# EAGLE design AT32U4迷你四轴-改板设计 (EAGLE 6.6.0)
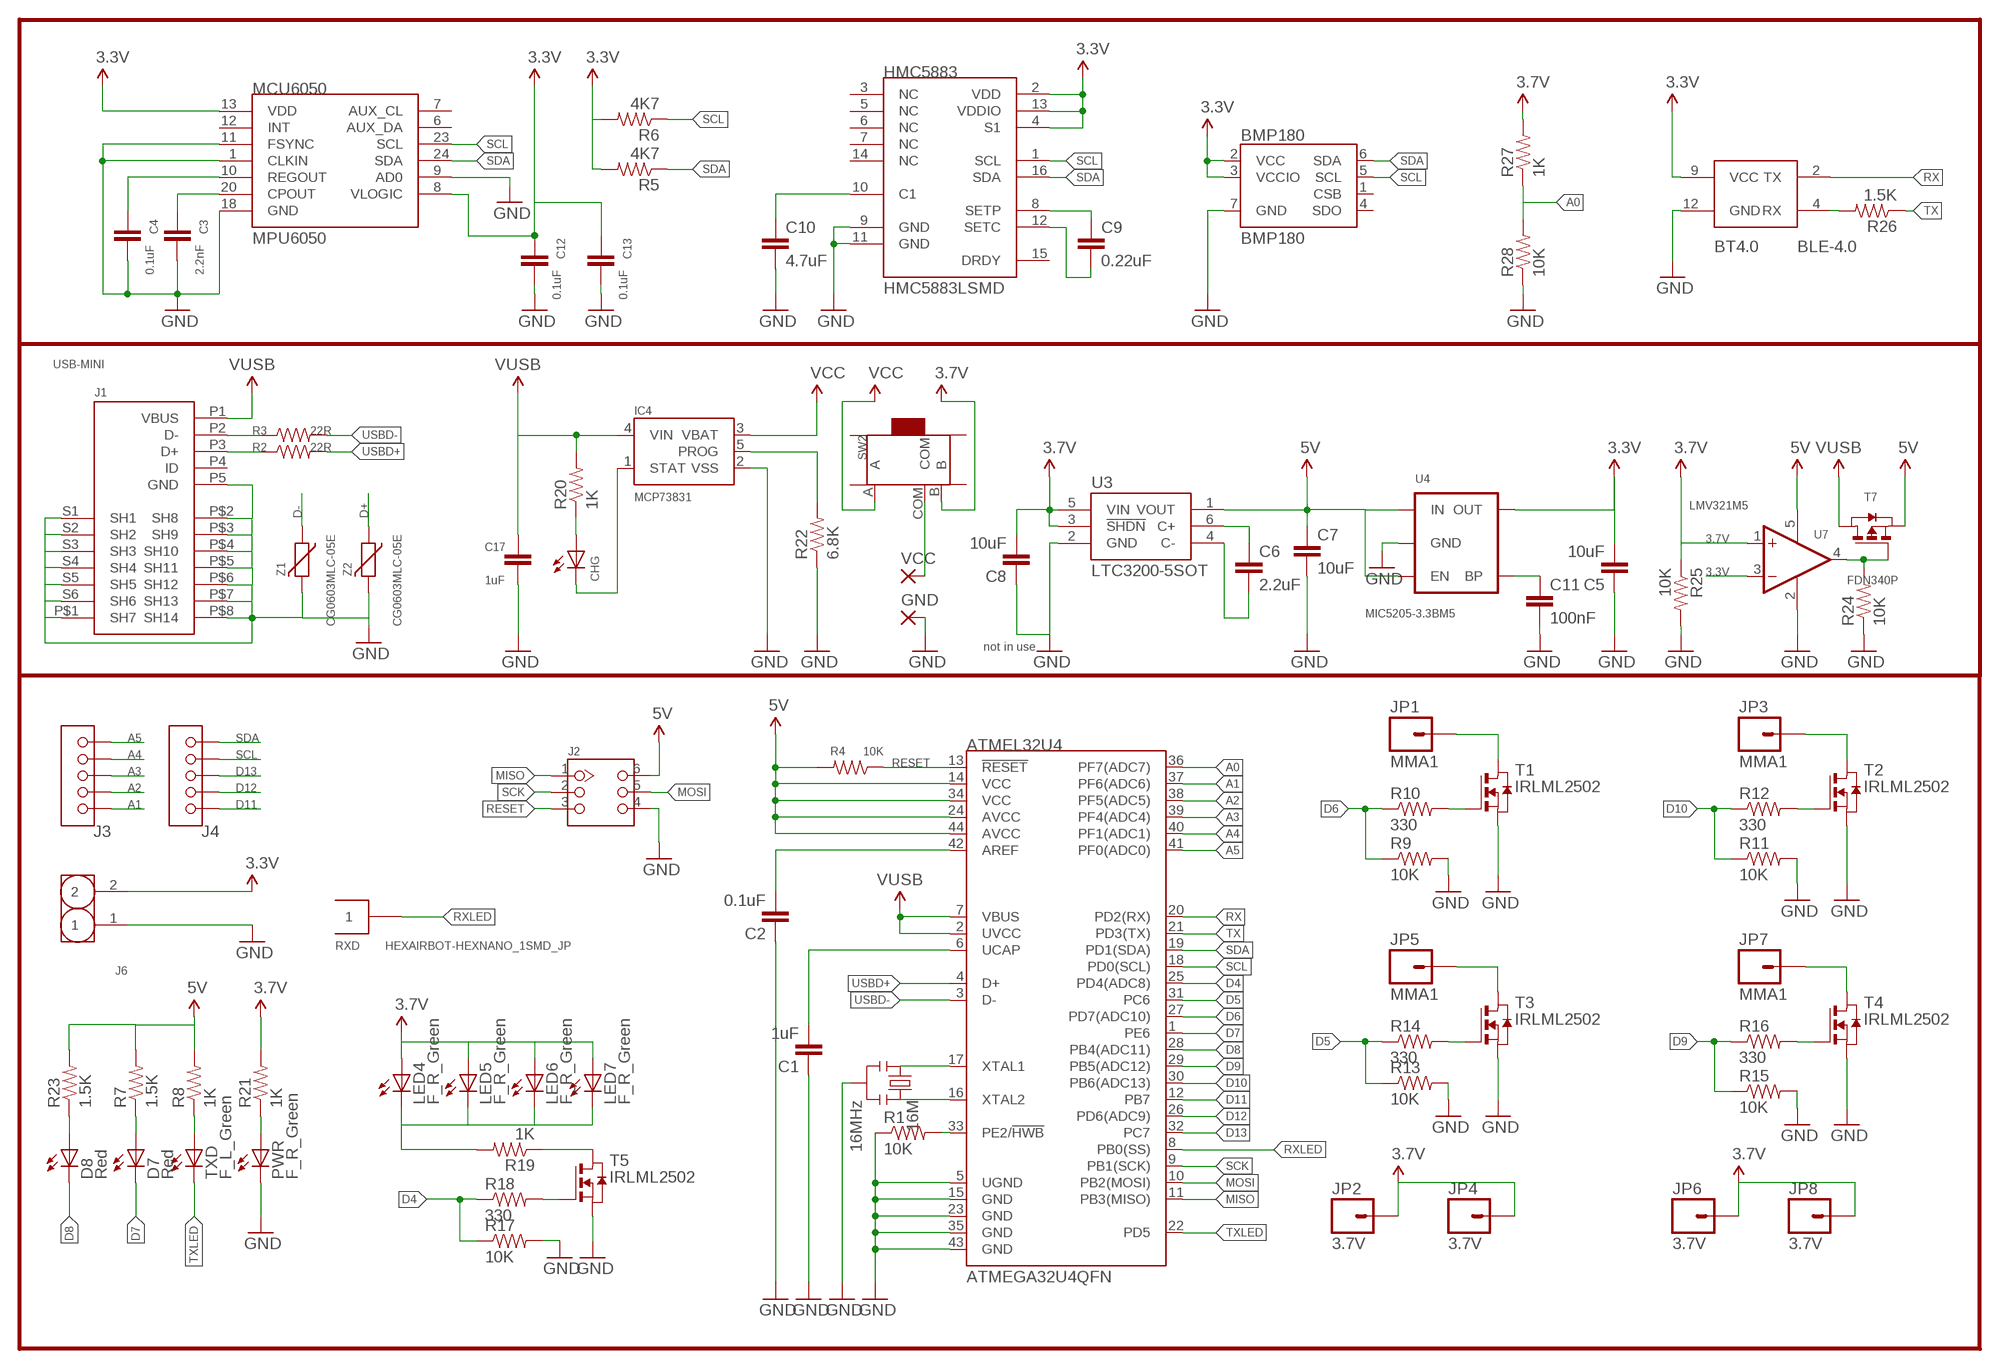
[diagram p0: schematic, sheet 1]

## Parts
16M  16MHz  RESONATOR16MHZ  [RESONATOR-SMD]
ATMEL32U4  ATMEGA32U4QFN  [SPARKFUN-DIGITALIC_QFN-44]
BMP180  BMP180  [BMP180]
BT4.0  BLE-4.0  HEXAIRBOT-HEXNANO_BLUETOOTH_HM11  [HEXAIRBOT-HEXNANO_BLUETOOTH_HM11]
C1  1uF  CAP0402-CAP  [0402-CAP]
C2  0.1uF  CAP0402-CAP  [0402-CAP]
C3  2.2nF  CAP0402-CAP  [0402-CAP]
C4  0.1uF  CAP0402-CAP  [0402-CAP]
C5  10uF  CAP0402-CAP  [0402-CAP]
C6  2.2uF  CAP0603-CAP  [0603-CAP]
C7  10uF  CAP0603-CAP  [0603-CAP]
C8  10uF  CAP0805  [0805]
C9  0.22uF  CAP0402-CAP  [0402-CAP]
C10  4.7uF  CAP0402-CAP  [0402-CAP]
C11  100nF  CAP0603-CAP  [0603-CAP]
C12  0.1uF  CAP0402-CAP  [0402-CAP]
C13  0.1uF  CAP0402-CAP  [0402-CAP]
C17  1uF  CAP0805  [0805]
CHG  Yellow  LEDCHIPLED_0603  [CHIPLED_0603]
D7  Red  LEDCHIPLED_0603  [CHIPLED_0603]
D8  Red  LEDCHIPLED_0603  [CHIPLED_0603]
GND  2,15/1,0  [2,15/1,0]
HMC5883  HMC5883LSMD  [16LPCC]
IC4  MCP73831  [SOT23-5]
J1  USB-MINI  [USB_MICRO]
J2  HEADER-2X3P-2.0  [2X3P-2.0]
J3  HEADER-5P-2.0  [5P-2.0]
J4  HEADER-5P-2.0  [5P-2.0]
J6  HEADER-2P-2.0  [2P-2.0]
JP1  MMA1  M01SMD-4.5X1.5  [PAD-1.5X4.5]
JP2  3.7V  M01SMD-4.5X1.5  [PAD-1.5X4.5]
JP3  MMA1  M01SMD-4.5X1.5  [PAD-1.5X4.5]
JP4  3.7V  M01SMD-4.5X1.5  [PAD-1.5X4.5]
JP5  MMA1  M01SMD-4.5X1.5  [PAD-1.5X4.5]
JP6  3.7V  M01SMD-4.5X1.5  [PAD-1.5X4.5]
JP7  MMA1  M01SMD-4.5X1.5  [PAD-1.5X4.5]
JP8  3.7V  M01SMD-4.5X1.5  [PAD-1.5X4.5]
LED4  F_R_Green  LEDCHIPLED_0603  [CHIPLED_0603]
LED5  F_R_Green  LEDCHIPLED_0603  [CHIPLED_0603]
LED6  F_R_Green  LEDCHIPLED_0603  [CHIPLED_0603]
LED7  F_R_Green  LEDCHIPLED_0603  [CHIPLED_0603]
MCU6050  MPU6050  TESTING_MPU-6050-1  [TESTING_QFN-24-4MM2]
PWR  F_R_Green  LEDCHIPLED_0603  [CHIPLED_0603]
R1  10K  RESISTOR0402-RES  [0402-RES]
R2  22R  RESISTOR0402-RES  [0402-RES]
R3  22R  RESISTOR0402-RES  [0402-RES]
R4  10K  RESISTOR0402-RES  [0402-RES]
R5  4K7  RESISTOR0402-RES  [0402-RES]
R6  4K7  RESISTOR0402-RES  [0402-RES]
R7  1.5K  RESISTOR0402-RES  [0402-RES]
R8  1K  RESISTOR0402-RES  [0402-RES]
R9  10K  RESISTOR0402-RES  [0402-RES]
R10  330  RESISTOR0402-RES  [0402-RES]
R11  10K  RESISTOR0402-RES  [0402-RES]
R12  330  RESISTOR0402-RES  [0402-RES]
R13  10K  RESISTOR0402-RES  [0402-RES]
R14  330  RESISTOR0402-RES  [0402-RES]
R15  10K  RESISTOR0402-RES  [0402-RES]
R16  330  RESISTOR0402-RES  [0402-RES]
R17  10K  RESISTOR0402-RES  [0402-RES]
R18  330  RESISTOR0402-RES  [0402-RES]
R19  1K  RESISTOR0402-RES  [0402-RES]
R20  1K  RESISTOR0402-RES  [0402-RES]
R21  1K  RESISTOR0402-RES  [0402-RES]
R22  6.8K  RESISTOR0402-RES  [0402-RES]
R23  1.5K  RESISTOR0402-RES  [0402-RES]
R24  10K  RESISTOR0402-RES  [0402-RES]
R25  10K  RESISTOR0402-RES  [0402-RES]
R26  1.5K  RESISTOR0402-RES  [0402-RES]
R27  1K  RESISTOR0402-RES  [0402-RES]
R28  10K  RESISTOR0402-RES  [0402-RES]
RXD  HEXAIRBOT-HEXNANO_1SMD_JP  [HEXAIRBOT-HEXNANO_1SMD]
SW2  SWITCH-3P-SMD-6.6X2.8  [3P-SMD-2CH-6.6X2.8-REINFORCE]
T1  IRLML2502  NMOSSOT23  [SOT-23]
T2  IRLML2502  NMOSSOT23  [SOT-23]
T3  IRLML2502  NMOSSOT23  [SOT-23]
T4  IRLML2502  NMOSSOT23  [SOT-23]
T5  IRLML2502  NMOSSOT23  [SOT-23]
T7  FDN340P  [SOT23]
TXD  F_L_Green  LEDCHIPLED_0603  [CHIPLED_0603]
U3  LTC3200-5SOT  [SOT23-6]
U4  MIC5205-3.3BM5  MIC52053.3V  [SOT23-5]
U7  LMV321M5  [SOT23-5]
VCC  2,15/1,0  [2,15/1,0]
Z1  CG0603MLC-05E  VARISTORCN0603  [CT/CN0603]
Z2  CG0603MLC-05E  VARISTORCN0603  [CT/CN0603]

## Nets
3.3V: BMP180.2(VCC) BMP180.3(VCCIO) BT4.0.9(VCC) C5.2 C12.1 C13.1 HMC5883.2(VDD) HMC5883.4(S1) HMC5883.13(VDDIO) J6.2 MCU6050.8(VLOGIC) MCU6050.13(VDD) R5.2 R6.2 U4.5(OUT) U7.3(-IN)
3.7V: C8.2 JP2.P$1 JP4.P$1 JP6.P$1 JP8.P$1 LED4.A LED5.A LED6.A LED7.A R21.2 R25.1 R27.2 SW2.B U3.3(!SHDN) U3.5(VIN) U7.1(+IN)
5V: ATMEL32U4.14(VCC) ATMEL32U4.24(AVCC) ATMEL32U4.34(VCC) ATMEL32U4.44(AVCC) C7.1 J2.6 R4.2 R7.2 R8.2 R23.2 T7.2(S) U3.1(VOUT) U4.1(IN) U4.3(EN) U7.5(V+)
A0: ATMEL32U4.36(PF7(ADC7)) R27.1 R28.2
A1: ATMEL32U4.37(PF6(ADC6)) J3.1
A2: ATMEL32U4.38(PF5(ADC5)) J3.2
A3: ATMEL32U4.39(PF4(ADC4)) J3.3
A4: ATMEL32U4.40(PF1(ADC1)) J3.4
A5: ATMEL32U4.41(PF0(ADC0)) J3.5
D4: ATMEL32U4.25(PD4(ADC8)) R17.1 R18.1
D5: ATMEL32U4.31(PC6) R13.1 R14.1
D6: ATMEL32U4.27(PD7(ADC10)) R9.1 R10.1
D7: ATMEL32U4.1(PE6) D7.C
D8: ATMEL32U4.28(PB4(ADC11)) D8.C
D9: ATMEL32U4.29(PB5(ADC12)) R15.1 R16.1
D10: ATMEL32U4.30(PB6(ADC13)) R11.1 R12.1
D11: ATMEL32U4.12(PB7) J4.1
D12: ATMEL32U4.26(PD6(ADC9)) J4.2
D13: ATMEL32U4.32(PC7) J4.3
D+: J1.P3(D+) R2.1 Z2.1
D-: J1.P2(D-) R3.1 Z1.1
GND: 16M.2 ATMEL32U4.5(UGND) ATMEL32U4.15(GND) ATMEL32U4.23(GND) ATMEL32U4.35(GND) ATMEL32U4.43(GND) BMP180.7(GND) BT4.0.12(GND) C1.1 C2.1 C3.2 C4.2 C5.1 C7.2 C8.1 C10.2 C11.2 C12.2 C13.2 C17.1 GND.1(P) HMC5883.9(GND) HMC5883.11(GND) IC4.2(VSS) J1.P5(GND) J1.P$1(SH7) J1.P$2(SH8) J1.P$3(SH9) J1.P$4(SH10) J1.P$5(SH11) J1.P$6(SH12) J1.P$7(SH13) J1.P$8(SH14) J1.S1(SH1) J1.S2(SH2) J1.S3(SH3) J1.S4(SH4) J1.S5(SH5) J1.S6(SH6) J2.4 J6.1 MCU6050.1(CLKIN) MCU6050.9(AD0) MCU6050.11(FSYNC) MCU6050.18(GND) PWR.C R1.1 R9.2 R11.2 R13.2 R15.2 R17.2 R22.1 R24.1 R25.2 R28.1 T1.2(S) T2.2(S) T3.2(S) T4.2(S) T5.2(S) U3.2(GND) U4.2(GND) U7.2(V-) Z1.2 Z2.2
MISO: ATMEL32U4.11(PB3(MISO)) J2.1
MOSI: ATMEL32U4.10(PB2(MOSI)) J2.5
N$1: 16M.1 ATMEL32U4.17(XTAL1)
N$2: 16M.3 ATMEL32U4.16(XTAL2)
N$3: CHG.C IC4.1(STAT)
N$4: CHG.A R20.1
N$5: ATMEL32U4.6(UCAP) C1.2
N$6: ATMEL32U4.42(AREF) C2.2
N$7: R8.1 TXD.A
N$8: C4.1 MCU6050.10(REGOUT)
N$9: C3.1 MCU6050.20(CPOUT)
N$10: D7.A R7.1
N$11: ATMEL32U4.33(PE2/!HWB) R1.2
N$12: R18.2 T5.3(G)
N$13: PWR.A R21.1
N$14: R12.2 T2.3(G)
N$15: R10.2 T1.3(G)
N$16: JP1.P$1 T1.1(D)
N$17: JP3.P$1 T2.1(D)
N$18: R14.2 T3.3(G)
N$19: JP5.P$1 T3.1(D)
N$20: R16.2 T4.3(G)
N$21: JP7.P$1 T4.1(D)
N$22: R19.1 T5.1(D)
N$23: C9.1 HMC5883.8(SETP)
N$24: LED4.C LED5.C LED6.C LED7.C R19.2
N$25: C6.1 U3.6(C+)
N$26: IC4.5(PROG) R22.2
N$27: C6.2 U3.4(C-)
N$28: C9.2 HMC5883.12(SETC)
N$29: C10.1 HMC5883.10(C1)
N$30: SW2.COM VCC.1(P)
N$31: C11.1 U4.4(BP)
N$32: D8.A R23.1
N$34: R24.2 T7.3(G) U7.4(OUT)
N$35: BT4.0.4(RX) R26.2
RESET: ATMEL32U4.13(!RESET) J2.3 R4.1
RX: ATMEL32U4.20(PD2(RX)) BT4.0.2(TX)
RXLED: ATMEL32U4.8(PB0(SS)) RXD.1
SCK: ATMEL32U4.9(PB1(SCK)) J2.2
SCL: ATMEL32U4.18(PD0(SCL)) BMP180.5(SCL) HMC5883.1(SCL) J4.4 MCU6050.23(SCL) R6.1
SDA: ATMEL32U4.19(PD1(SDA)) BMP180.6(SDA) HMC5883.16(SDA) J4.5 MCU6050.24(SDA) R5.1
TX: ATMEL32U4.21(PD3(TX)) R26.1
TXLED: ATMEL32U4.22(PD5) TXD.C
USBD+: ATMEL32U4.4(D+) R2.2
USBD-: ATMEL32U4.3(D-) R3.2
VCC: IC4.3(VBAT) SW2.A
VUSB: ATMEL32U4.2(UVCC) ATMEL32U4.7(VBUS) C17.2 IC4.4(VIN) J1.P1(VBUS) R20.2 T7.1(D)
Unconnected: BMP180.1(CSB) BMP180.4(SDO) HMC5883.3(NC) HMC5883.5(NC) HMC5883.6(NC) HMC5883.7(NC) HMC5883.14(NC) HMC5883.15(DRDY) J1.P4(ID) MCU6050.6(AUX_DA) MCU6050.7(AUX_CL) MCU6050.12(INT) SW2.SS1 SW2.SS2 SW2.SS3 SW2.SS4

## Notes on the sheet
- not in use

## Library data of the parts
16M = SparkFun-FreqCtrl:RESONATOR: Resonator Small SMD resonator. Used, eg, on the Arduino Pro/ Pro Mini boards. 8MHz- XTAL-08895 16MHz- XTAL-08900; PROD_ID: XTAL-08900
ATMEL32U4 = SparkFun-DigitalIC:ATMEGA32U4: Atmel 44-pin 8-bit Microcontroller with 32KBytes of ISP Flash and USB Controller ----- Please use the QFN-44-NOPAD_1:1 package for the footprint of all boards using a 32U4. Route traces directly away from the pads as much as possible.
BMP180 = duinofun-ic:BMP180: BMP085 Pressure Sensor Great little MEMS pressure sensor. SKU: COM-09603
BT4.0 = MainBoard:HEXAIRBOT-HEXNANO_BLUETOOTH_HM11: BLE 4.0 Module
C1-C13 = SparkFun-Passives:CAP: Capacitor
C17 = SparkFun:CAP: Capacitor
CHG D7 D8 LED4-LED7 PWR TXD = led:LED: LED
GND VCC = wirepad:2,15/1,0: THROUGH-HOLE PAD
HMC5883 = HexAirbot-HexNano:HMC5883L: 3 Axis Digital Compass IC
IC4 = SparkFun:MCP73831: Microchip's MCP73831 Miniature single cell, fully integrated Li-Ion, Li-polymer charge management controller http://ww1.microchip.com/downloads/en/DeviceDoc/21984a.pdf
J1 = QXZ:USB-MINI
J2 = SeeedStudio-Connector:HEADER-2X3P
J3 J4 = SeeedStudio-Connector:HEADER-5P
J6 = SeeedStudio-Connector:HEADER-2P
JP1-JP8 = SparkFun-Connectors:M01: Header 1
MCU6050 = MPU6050:TESTING_MPU-6050
R1-R28 = SparkFun-Passives:RESISTOR: Resistor
RXD = MainBoard:HEXAIRBOT-HEXNANO_1SMD_JP
SW2 = duinofun-ic:SWITCH-3P-SMD
T1-T5 = zetex:NMOSSOT23: MOS FET; OC_FARNELL: unknown; OC_NEWARK: unknown
T7 = HexAirbot-HexNano:FDN340P: MOS FET
U3 = HexAirbot-HexNano:LTC3200-5: Linear Technology. Low Noise, Regulated Charge Pump DC/DC Converters, SOT23-6. Fixed 5V ± 4% Output or ADJ VIN Range: 2.7V to 4.5V
U4 = SparkFun-PowerIC:MIC5205: MIC5205 150mA vreg 3.3V - VREG-00822 5V - VREG-00823; PROD_ID: VREG-00822
U7 = linear:LMV321?*: General Purpose, Low Voltage, Rail-to-Rail Output Operational Amplifiers Source: http://www.national.com/mpf/LM/LMV321.html http://www.national.com/dt/lmv_qual.pdf
Z1 Z2 = varistor:VARISTOR: VARISTOR

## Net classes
0 default: width 0.254 mm, drill 0.61 mm, clearance 0.254 mm
2 gnd: width 0.254 mm, drill 0.61 mm, clearance 0.254 mm

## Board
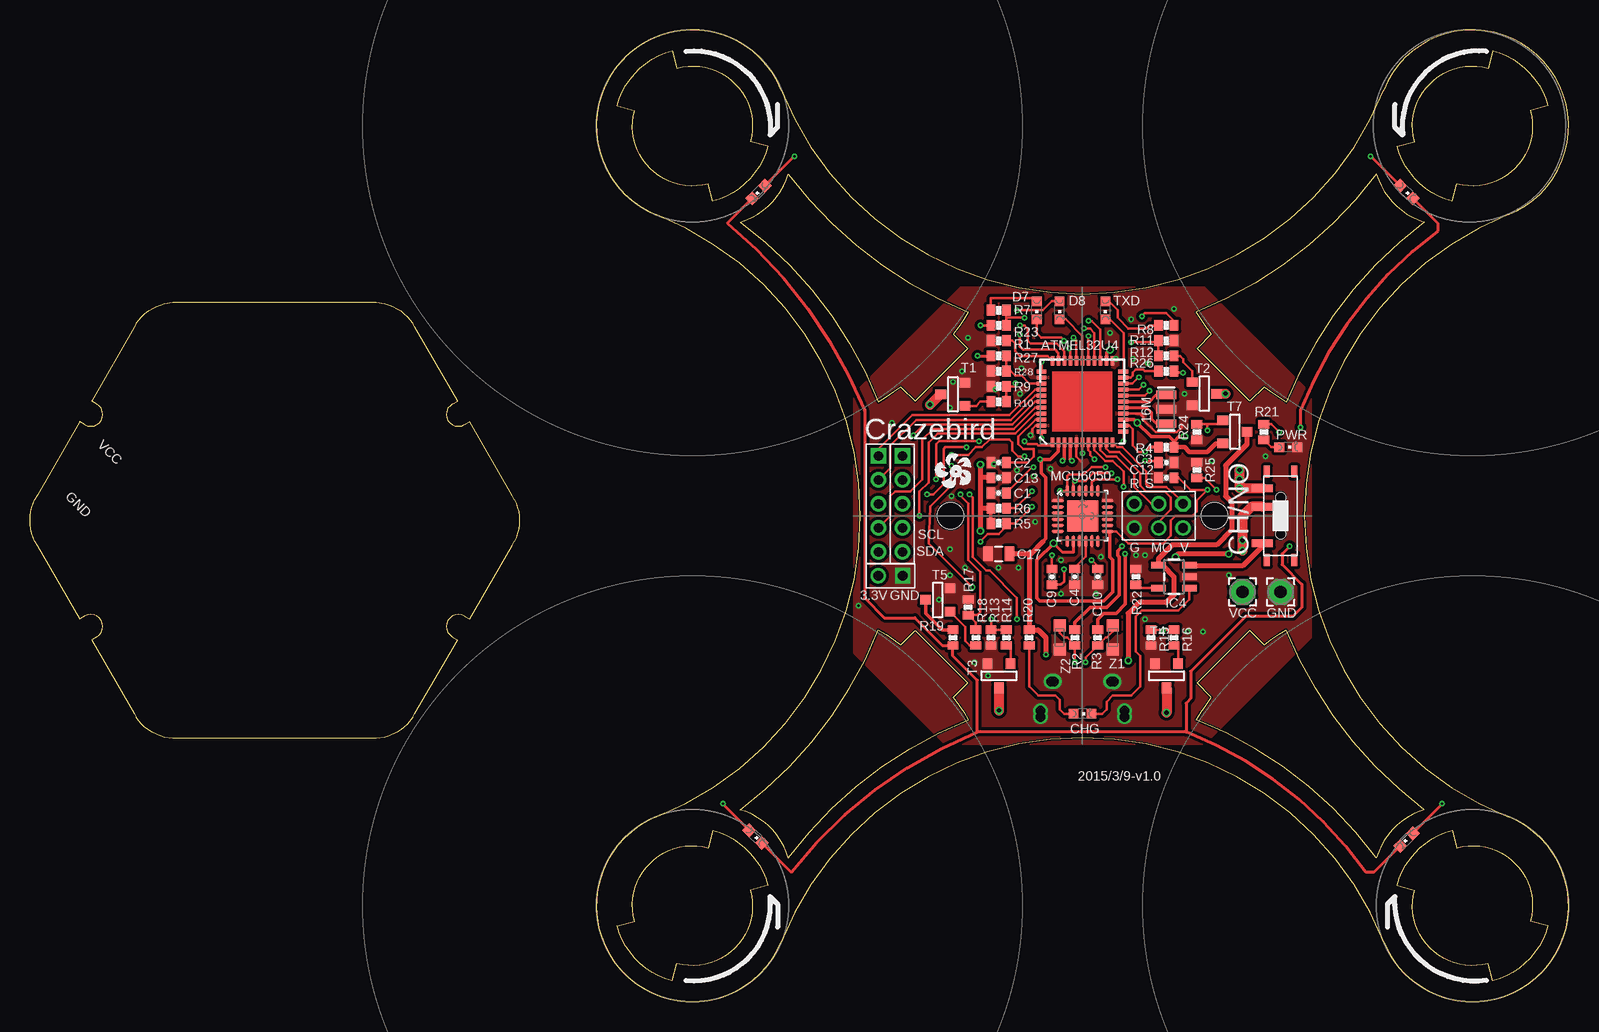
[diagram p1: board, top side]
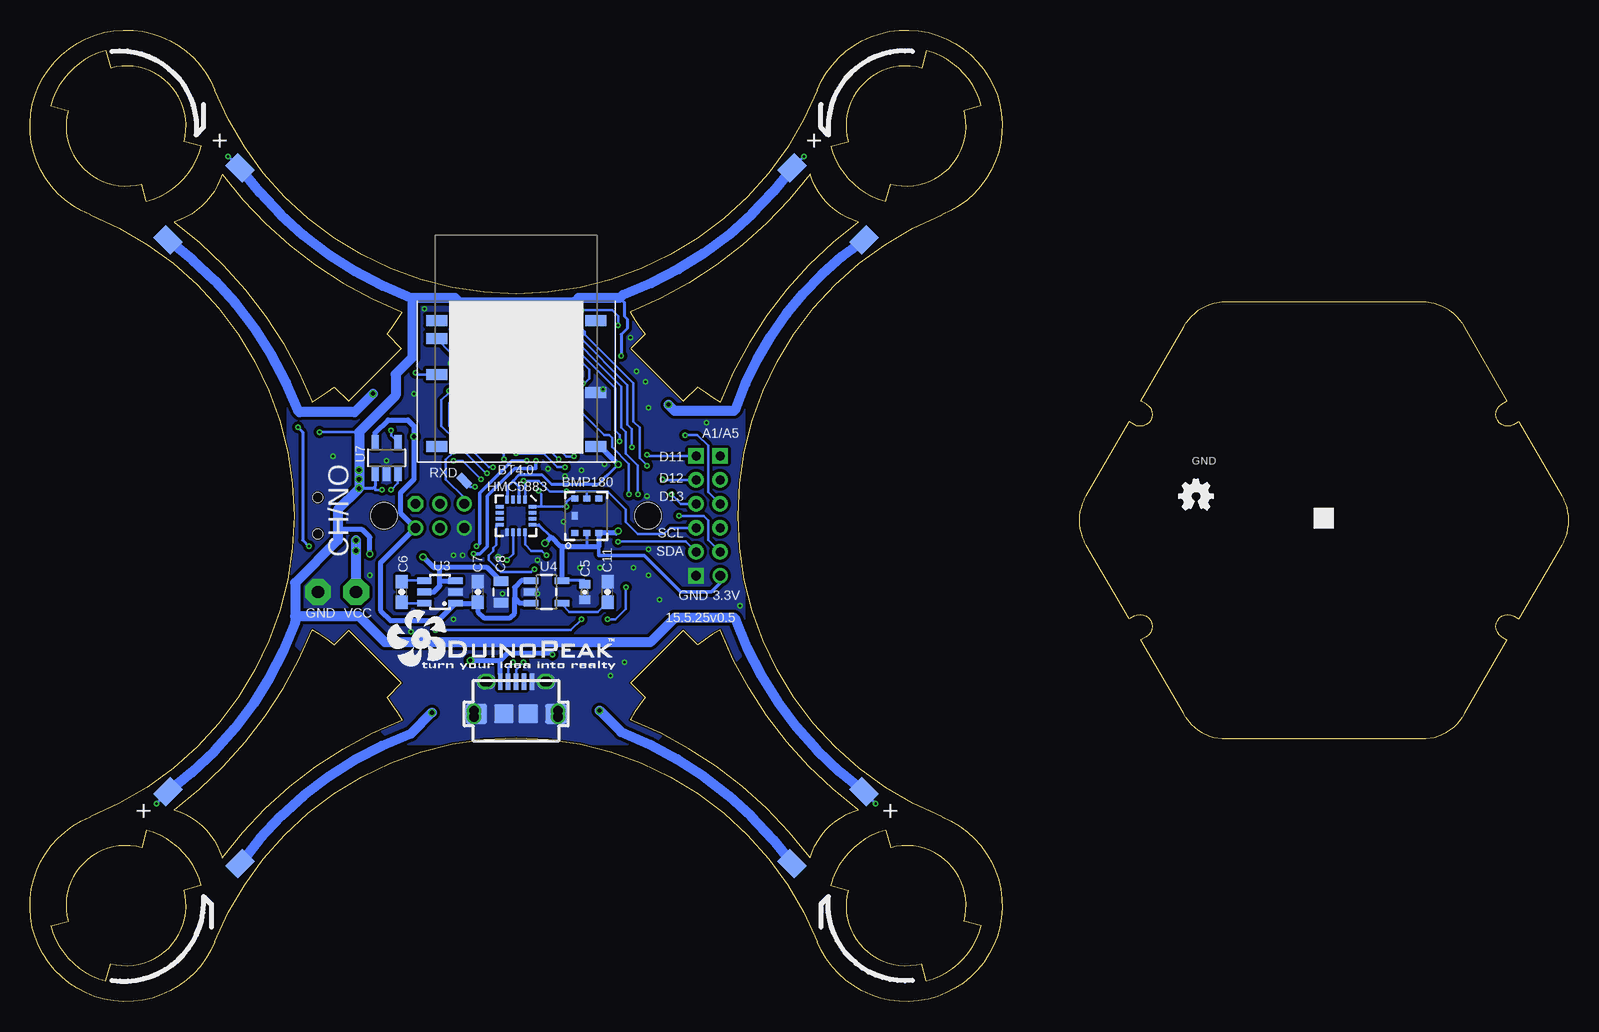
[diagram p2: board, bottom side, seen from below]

Size 128.21 x 81.01 mm. Coordinates in mm from the lower left corner, seen from the top.
Outline: 124 segments
Copper layers (1*16): Top 0.035mm / dielectric 1.5mm / Bottom 0.035mm
Design rules "Sparkfun *": minimum track width 5mil, minimum drill 8mil, track to track 5mil, track to pad 5mil, pad to pad 8mil, via to via 8mil, smd to smd 5mil, copper to edge 5mil, drill to drill 8mil, minimum pad ring 7mil, minimum via ring 5mil, stop-mask expansion 4mil, vias tented up to drill 25mil, thermal gap 5mil

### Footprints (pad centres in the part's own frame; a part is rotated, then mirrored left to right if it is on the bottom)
RESONATOR-SMD = smd 0.7 x 1.7: 1 -1.2,0; 2 0,0; 3 1.2,0
SPARKFUN-DIGITALIC_QFN-44 = smd 0.8 x 0.3: 1 -3.4,2.5; 2 -3.4,2; 3 -3.4,1.5; 4 -3.4,1; 5 -3.4,0.5; 6 -3.4,0; 7 -3.4,-0.5; 8 -3.4,-1; 9 -3.4,-1.5; 10 -3.4,-2; 11 -3.4,-2.5; 23 3.4,-2.5; 24 3.4,-2; 25 3.4,-1.5; 26 3.4,-1; 27 3.4,-0.5; 28 3.4,0; 29 3.4,0.5; 30 3.4,1; 31 3.4,1.5; 32 3.4,2; 33 3.4,2.5 | smd 0.3 x 0.8: 12 -2.5,-3.4; 13 -2,-3.4; 14 -1.5,-3.4; 15 -1,-3.4; 16 -0.5,-3.4; 17 0,-3.4; 18 0.5,-3.4; 19 1,-3.4; 20 1.5,-3.4; 21 2,-3.4; 22 2.5,-3.4; 34 2.5,3.4; 35 2,3.4; 36 1.5,3.4; 37 1,3.4; 38 0.5,3.4; 39 0,3.4; 40 -0.5,3.4; 41 -1,3.4; 42 -1.5,3.4; 43 -2,3.4; 44 -2.5,3.4
BMP180 = smd 0.5 x 0.6: 1 -1.45,1.45; 2 -1.45,0.45; 3 -1.45,-0.55; 4 1.45,-0.55; 5 1.45,0.45; 6 1.45,1.45 | smd 0.6 x 0.5: 7 0,1.45
HEXAIRBOT-HEXNANO_BLUETOOTH_HM11 = smd 1.75 x 0.9: 1 -6.625,4.859; 2 -6.625,3.359; 4 -6.625,0.359; 8 -6.625,-5.641; 9 6.625,-5.641; 12 6.625,-1.141; 16 6.625,4.859
0402-CAP = smd 0.7 x 0.9: 1 -0.65,0; 2 0.65,0
0603-CAP = smd 1.1 x 1: 1 -0.85,0; 2 0.85,0
0805 = smd 0.8 x 1.2: 1 -0.9,0; 2 0.9,0
CHIPLED_0603 = smd 0.8 x 0.8: A 0,-0.75; C 0,0.75
2,15/1,0 = drill 1.016 pad 2.159 octagon: 1 0,0
16LPCC = smd 0.65 x 0.28: 1 -1.37,0.75; 2 -1.37,0.25; 3 -1.37,-0.25; 4 -1.37,-0.75; 9 1.37,-0.75; 10 1.37,-0.25; 11 1.37,0.25; 12 1.37,0.75 | smd 0.28 x 0.65: 5 -0.75,-1.37; 6 -0.25,-1.37; 7 0.25,-1.37; 8 0.75,-1.37; 13 0.75,1.37; 14 0.25,1.37; 15 -0.25,1.37; 16 -0.75,1.37
SOT23-5 = smd 0.55 x 1.2: 1 -0.95,-1.3; 2 0,-1.3; 3 0.95,-1.3; 4 0.95,1.3; 5 -0.95,1.3
USB_MICRO = smd 0.406 x 1.346: P1 -1.321,2.692; P2 -0.66,2.692; P3 0,2.692; P4 0.66,2.692; P5 1.321,2.692 | drill 0.8 pad 1.27: P$1 -2.616,2.692 | drill 0.8 pad 1.245: P$2 -2.362,2.692; P$7 2.362,2.692; P$8 2.616,2.692 | drill 0.8 pad 1.143: P$3 -3.505,-0.254; P$4 -3.505,0.254; P$5 3.505,0.254; P$6 3.505,-0.254 | smd 1.778 x 1.651: S1 -3.302,0; S2 3.302,0 | smd 1.524 x 1.27: S3 -2.489,2.692; S4 2.489,2.692 | smd 1.626 x 1.524: S5 -1.016,0; S6 1.016,0
2X3P-2.0 = drill 0.813 pad 1.27 octagon: 1 -1.016,2.032 | drill 0.813 pad 1.27: 2 -1.016,0; 3 -1.016,-2.032; 4 1.016,-2.032; 5 1.016,0; 6 1.016,2.032
5P-2.0 = drill 0.762 pad 1.27 square: 1 0,4 | drill 0.762 pad 1.27: 2 0,2; 3 0,0; 4 0,-2; 5 0,-4
2P-2.0 = drill 0.813 pad 1.27 square: 1 -1.016,0 | drill 0.813 pad 1.27: 2 1.016,0
PAD-1.5X4.5 = smd 1.5 x 2: P$1 0,0
TESTING_QFN-24-4MM2 = smd 1.016 x 0.254: 1 -2.066,1.257; 2 -2.066,0.75; 3 -2.066,0.247; 4 -2.066,-0.287; 5 -2.066,-0.792; 6 -2.066,-1.297; 13 2.086,-1.297; 14 2.086,-0.792; 15 2.086,-0.287; 16 2.086,0.247; 17 2.086,0.75; 18 2.086,1.257 | smd 0.254 x 1.016: 7 -1.267,-2.122; 8 -0.762,-2.122; 9 -0.258,-2.122; 10 0.278,-2.122; 11 0.78,-2.122; 12 1.287,-2.122; 19 1.287,2.082; 20 0.78,2.082; 21 0.278,2.082; 22 -0.258,2.082; 23 -0.762,2.082; 24 -1.267,2.082 | smd 2.616 x 2.616: P$1 0.02,-0.01
0402-RES = smd 0.7 x 0.9: 1 -0.65,0; 2 0.65,0
HEXAIRBOT-HEXNANO_1SMD = smd 1.27 x 0.635: 1 0,0
3P-SMD-2CH-6.6X2.8-REINFORCE = smd 1.778 x 0.635: A 1.524,2.286; B 1.524,-2.286; COM 1.524,-0.762 | smd 0.508 x 1.016: SS1 -1.143,-3.683; SS2 1.143,-3.683; SS3 1.143,3.683; SS4 -1.143,3.683 | hole 0.813: 0,-1.524; 0,1.524
SOT-23 = smd 0.787 x 0.889: 1 0.025,-1.016; 2 -0.94,1.016; 3 0.991,1.016
SOT23 = smd 0.787 x 0.889: 1 0.025,-1.016; 2 -0.94,1.016; 3 0.991,1.016
SOT23-6 = smd 0.55 x 1.2: 1 -0.95,-1.3; 2 0,-1.3; 3 0.95,-1.3; 4 0.95,1.3; 5 0,1.3; 6 -0.95,1.3
SOT23-5' = smd 0.6 x 1.2: 1 -0.95,-1.306; 2 0,-1.306; 3 0.95,-1.306; 4 0.95,1.306; 5 -0.95,1.306
XFK-MINI-X4B = hole 2.2: -11,0; 11,0
CT/CN0603 = smd 1 x 1: 1 -1,0; 2 1,0

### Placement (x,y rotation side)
16M  94.69,49.4 270 top
ATMEL32U4  87.71,50.03 90 top
BMP180  81.36,40.51 90 bottom
BT4.0  87.71,51.94 0 bottom
C1  80.72,42.41 0 top
C2  80.72,44.95 0 top
C3  94.69,44.95 0 top
C4  87.07,35.43 270 top
C5  81.99,34.16 90 bottom
C6  97.23,34.16 90 bottom
C7  90.88,34.16 90 bottom
C8  88.98,34.16 90 bottom
C9  85.17,35.43 90 top
C10  88.98,35.43 270 top
C11  80.09,34.16 90 bottom
C12  94.69,43.68 180 top
C13  80.72,43.68 0 top
C17  80.72,37.33 0 top
CHG  87.71,24 270 top
D7  83.9,57.65 180 top
D8  85.8,57.65 180 top
GND  104.22,34.16 0 top
HMC5883  87.71,40.51 270 bottom
IC4  95.33,35.43 90 top
J1  87.71,24 0 bottom
J2  94.06,40.51 270 top
J3  70.71,41.51 0 top
J4  72.71,41.51 0 top
J6  71.71,35.51 180 top
JP1  58.71,63.51 135 bottom
JP2  64.71,69.51 135 bottom
JP3  116.71,63.51 45 bottom
JP4  116.71,17.51 315 bottom
JP5  64.71,11.51 45 bottom
JP6  110.71,69.51 45 bottom
JP7  110.71,11.51 315 bottom
JP8  58.71,17.51 45 bottom
LED4  60.71,67.51 135 top
LED5  114.71,67.51 225 top
LED6  114.71,13.51 135 top
LED7  60.46,13.75 225 top
MCU6050  87.71,40.51 0 top
PWR  104.85,46.22 270 top
R1  80.72,55.11 0 top
R2  87.07,30.35 90 top
R3  88.98,30.35 90 top
R4  94.69,46.22 0 top
R5  80.72,39.87 180 top
R6  80.72,41.14 180 top
R7  80.72,57.65 0 top
R8  94.69,56.38 0 top
R9  80.72,51.3 180 top
R10  80.72,50.03 180 top
R11  94.69,55.11 0 top
R12  94.69,53.84 0 top
R13  80.09,30.35 270 top
R14  81.36,30.35 270 top
R15  93.42,30.35 270 top
R16  95.33,30.35 270 top
R17  78.18,32.89 90 top
R18  78.82,30.35 270 top
R19  76.91,30.35 270 top
R20  83.26,30.35 90 top
R21  102.82,47.49 90 top
R22  92.15,35.43 270 top
R23  80.72,56.38 0 top
R24  97.23,47.49 90 top
R25  97.23,44.32 90 top
R26  94.69,52.57 0 top
R27  80.72,53.84 180 top
R28  80.72,52.57 0 top
RXD  92.02,43.43 315 bottom
SW2  104.22,40.51 180 top
T1  76.91,50.67 270 top
T2  97.87,50.67 90 top
T3  80.72,27.17 0 top
T4  94.69,27.17 0 top
T5  75.64,33.52 270 top
T7  100.41,47.49 90 top
TXD  89.61,57.65 180 top
U3  94.06,34.16 90 bottom
U4  85.17,34.16 270 bottom
U7  LMV321M5  [SOT23-5']  98.5,45.33 0 bottom
U$1  [OSHW_FILLX100_NOTEXT]  32.46,41.01 0 bottom
U$2  [DUINOFUN-LOGO-0.65]  98.5,27.68 0 bottom
U$3  [DUINOFUN-LOGO-PCB-0.4]  75.39,42.79 0 top
U$5  [XFK-MINI-X4B]  87.71,40.51 0 top
VCC  101.04,34.16 0 top
Z1  90.25,30.35 270 top
Z2  85.8,30.35 270 top

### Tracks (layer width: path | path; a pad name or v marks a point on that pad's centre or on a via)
3.3V  (via drill 0.2, 0.36)
  Top 0.203: 80.09,41.14 79.2,41.14 | MCU6050.13 90.53,39.21 91.52,38.22 94.44,38.22 95.07,38.86 95.07,40.13 95.45,40.51 96.85,40.51 97.23,40.89 97.23,41.78 v98.12,42.67 96.72,42.67 95.71,43.68 C12.1
  Top 0.254: MCU6050.8 86.94,37.46 86.06,37.46 v85.29,38.22
  Top 0.305: R5.2 R6.2 80.09,41.14 | 80.09,41.14 | 80.09,41.14 | v85.29,38.22 83.9,36.82 83.9,33.65 84.15,33.39 89.48,33.39 90.25,34.16 90.25,36.82 89.99,37.08 89.99,39.01 MCU6050.13
  Top 0.406: C13.1 79.2,43.68 | 79.2,43.68 79.2,41.14 | 79.2,41.14 R6.2 | v79.2,44.79 79.2,43.68 | 79.2,41.14 v79.2,39.24
  Bottom 0.203: BT4.0.9 80.71,46.3 | U7.3 97.55,43.23 v98.12,42.67
  Bottom 0.254: HMC5883.2 87.46,42.92 87.96,43.42 87.96,43.43 | HMC5883.4 88.46,42.93 87.96,43.43 | HMC5883.13 85.81,39.76 84.79,38.73 | 84.02,37.97 83.87,37.97 | BMP180.2 81.81,37.97 | C5.2 81.99,35.11 U4.5 | v79.2,44.79 80.07,43.91 80.33,43.68 80.83,43.17 84.79,43.17 85.55,43.94 87.45,43.94 87.96,43.43
  Bottom 0.305: J6.2 70.69,34.92 71.45,34.16 73.99,34.16 77.04,37.2 80.81,37.2 80.81,37.97
  Bottom 0.406: 84.02,37.97 84.79,38.73 v85.29,38.22 | U4.5 83.87,37.97 81.81,37.97 80.81,37.97 BMP180.3 79.38,39.06 v79.2,39.24 | 80.71,46.3 v79.2,44.79
3.7V  (via drill 0.2, 0.36)
  Top 0.203: v104.09,47.49 103.44,48.14 R21.2 | R25.1 97.88,43.67 v98.88,42.67
  Top 0.254: LED7.A 57.73,16.48 v57.73,16.5 | LED4.A 63.68,70.48 v63.7,70.48 | LED6.A 117.68,16.48 v117.68,16.5 | LED5.A 111.73,70.48 v111.71,70.48 | v78.94,53.84 R27.2
  Top 0.406: v99.9,37.33 95.71,37.33 v95.45,37.08
  Top 0.813: SW2.B v100.79,42.79 v100.79,43.55 v100.79,44.32
  Bottom 0.203: 100.79,47.49 v104.09,47.49 | 99.45,42.99 99.45,42.67 v98.88,42.67
  Bottom 0.254: v57.73,16.5 58.71,17.48 JP8.P$1 | v63.7,70.48 64.68,69.51 JP2.P$1 | v117.68,16.5 116.71,17.48 JP4.P$1 | v111.71,70.48 110.74,69.51 JP6.P$1 | U7.1 99.45,42.99 99.64,42.79 v100.79,42.79 | 79.07,58.67 78.69,58.29 78.69,57.14 78.44,56.89 78.44,56.13 78.94,55.62 v78.94,53.84
  Bottom 0.406: U3.5 94.56,34.16 94.06,34.66 94.06,35.05 | C8.2 90.11,36.19 94.06,36.19 | 100.72,42.79 v100.79,42.79 | v99.9,37.33 99.9,38.73 100.53,39.36 102.44,39.36 102.57,39.24 | 94.06,36.19 94.56,36.19 v95.45,37.08 | 94.06,35.05 94.06,36.19 | U3.3 92.82,35.05 94.06,35.05
  Bottom 0.813: 106.12,32.12 106.12,34.92 102.57,38.47 102.57,39.24 102.57,41.01 v100.79,42.79 100.79,47.49 97.74,50.54 97.74,52.32 96.34,53.71 96.34,58.54 96.47,58.67 | 106.12,32.12 106.12,31.62 arc34 JP4.P$1 | JP2.P$1 arc34 78.82,58.92 79.07,58.67 82.5,58.67 82.88,58.29 92.41,58.29 92.79,58.67 96.47,58.67 | 96.47,58.67 arc33 JP6.P$1 | JP8.P$1 arc33 69.42,31.87 69.55,32 74.5,32 76.53,29.97 98.63,29.97 100.79,32.12 106.12,32.12
5V  (via drill 0.2, 0.36)
  Top 0.203: 81.37,57.02 R23.2 | ATMEL32U4.34 84.31,53.3 v84.28,53.33 | R7.2 81.37,57.02 | 81.37,57.02 v82.88,57.02 | v92.66,57.14 92.91,57.4 94.69,57.4 95.34,56.75 R8.2
  Top 0.305: ATMEL32U4.24 89.74,53.84 89.74,54.13 89.96,54.35 v89.99,54.35 | ATMEL32U4.14 92,48.53 92.28,48.38 v92.28,48.25 93.42,47.11 94.95,47.11 95.34,46.71 | 95.34,46.71 R4.2 | 95.34,46.71 95.74,47.11 v96.22,47.11 | ATMEL32U4.44 84.28,47.53 v84.28,46.98
  Top 0.356: T7.2 98.83,46.55 98.12,45.84 96.6,45.84 96.22,46.22 R4.2
  Top 0.406: 95.34,46.49 R4.2
  Bottom 0.203: v82.88,57.02 83.9,57.02 84.4,57.52 92.28,57.52 v92.66,57.14 92.66,54.86 92.15,54.35 v89.99,54.35
  Bottom 0.305: v89.99,54.35 89.74,54.1 89.74,53.33 | 89.74,53.33 v84.28,53.33 84.28,48 | 89.74,53.33 91.52,51.56 91.52,48.25 | 84.28,48 v84.28,46.98 | 84.28,48 85.04,47.24 90.5,47.24 91.52,48.25 | 91.52,48.25 v92.28,48.25
  Bottom 0.406: U4.1 87.26,35.11 87.83,34.54 87.83,33.65 | U4.3 87.39,33.21 87.83,33.65 | U7.5 99.45,47.43 98.37,48.51 96.72,48.51 96.22,48 v96.22,47.11 96.22,43.55 97.36,42.41 97.36,40.76 J2.6 99.01,36.57 99.01,32.63 98.12,31.74 94.22,31.74 U3.1 90.98,33.21 C7.1 90.88,32.51 90.37,32 88.21,32 87.83,32.38 87.83,33.65
A0
  Top 0.203: R27.1 R28.2 81.74,52.57 82.12,52.19 82.63,52.19 83.29,51.53 ATMEL32U4.36
A1
  Top 0.203: J3.1 70.71,46.09 73.5,48.89 81.61,48.89 83.75,51.03 ATMEL32U4.37
A2
  Top 0.203: ATMEL32U4.38 83.76,50.53 81.74,48.51 73.86,48.51 71.7,46.35 71.7,44.5 J3.2
A3  (via drill 0.2)
  Top 0.203: ATMEL32U4.39 83.77,50.03 81.86,48.13 74.5,48.13 v73.61,47.24
  Bottom 0.203: J3.3 71.7,42.5 71.7,46.35 72.59,47.24 v73.61,47.24
A4
  Top 0.203: ATMEL32U4.40 83.78,49.53 81.99,47.75 75.26,47.75 74.37,46.86 74.37,43.55 73.36,42.54 72.09,42.54 71.7,42.16 71.7,40.5 J3.4
A5  (via drill 0.2)
  Top 0.203: ATMEL32U4.41 83.79,49.03 82.12,47.36 75.64,47.36 74.88,46.6 74.88,43.3 74.12,42.54 v74.12,40.51
  Bottom 0.203: v74.12,40.51 72.09,40.51 71.7,40.13 71.7,38.5 J3.5
D4  (via drill 0.2)
  Top 0.203: R18.1 78.82,31.6 R17.1 78.93,32.24 79.2,32.51 79.2,35.81 78.18,36.82 78.18,41.52 77.55,42.16 v77.55,42.28 | ATMEL32U4.25 89.21,56.02 88.47,56.76 v88.21,56.76
  Bottom 0.203: v77.55,42.28 77.55,44.7 78.56,45.71 78.56,47.49 78.94,47.87 78.94,51.3 84.53,56.89 88.09,56.89 v88.21,56.76
D5  (via drill 0.2)
  Top 0.203: ATMEL32U4.31 86.21,54.2 85.55,54.86 83.39,54.86 83.13,55.11 83.13,56.13 82.88,56.38 v82.5,56.38 | v80.09,31.87 R13.1 R14.1 | v78.56,34.54 74.88,38.22 75.01,41.27 76.78,43.05 v76.78,44.7
  Bottom 0.203: v82.5,56.38 81.99,55.87 81.99,55.62 77.93,51.56 77.93,48.38 77.42,47.87 77.42,45.33 v76.78,44.7 | v78.56,34.54 78.56,32.76 79.45,31.87 v80.09,31.87
D6  (via drill 0.2)
  Top 0.203: R10.1 R9.1 81.99,51.3 82.12,51.43 v82.12,51.56 | ATMEL32U4.27 88.21,55.48 v88.21,55.49
  Bottom 0.203: v88.21,55.49 87.71,55.49 87.07,56.13 85.04,56.13 81.61,52.7 81.61,51.94 81.99,51.56 v82.12,51.56
D7  (via drill 0.2)
  Top 0.203: D7.C 83.9,55.75 84.28,55.37 85.93,55.37 v86.18,55.11 | v82.88,46.73 83.13,46.48 83.9,46.48 84.02,46.35 84.92,46.35 ATMEL32U4.1 85.21,46.48
  Bottom 0.203: v86.18,55.11 85.29,55.11 83.77,53.59 83.77,49.9 82.88,49.02 v82.88,46.73
D8
  Top 0.203: ATMEL32U4.28 87.71,55.49 86.3,56.9 D8.C
D9  (via drill 0.2)
  Top 0.203: ATMEL32U4.29 87.21,55.1 v86.94,55.37 | v82.25,31.87 82.25,33.65 79.96,35.93 79.71,35.93 78.56,37.08 78.56,42.03 v78.31,42.28 | R16.1 95.31,30.98 v94.44,30.98 93.44,30.98 R15.1
  Bottom 0.203: v86.94,55.37 86.69,55.62 85.17,55.62 83.26,53.71 83.26,50.16 80.34,47.24 79.96,47.24 79.71,46.98 79.71,46.22 78.31,44.82 v78.31,42.28 | v82.25,31.87 83.13,30.98 v94.44,30.98
D10  (via drill 0.2)
  Top 0.203: R12.1 R11.1 93.91,54.98 v91.77,54.98 | ATMEL32U4.30 86.71,54.33 v86.56,54.48
  Bottom 0.203: v91.77,54.98 89.48,54.98 88.98,54.48 v86.56,54.48
D11  (via drill 0.2)
  Top 0.203: ATMEL32U4.12 91.14,47.5 v91.14,46.73 | v82.88,45.46 82.37,45.46 81.86,45.97 81.86,46.6 81.61,46.86 79.96,46.86 79.32,46.22 78.82,46.22 78.18,45.59 v76.78,45.59
  Bottom 0.203: J4.1 76.7,45.51 v76.78,45.59 | v82.88,45.46 83.52,45.46 83.9,45.84 84.15,45.84 85.04,46.73 v91.14,46.73
D12  (via drill 0.2)
  Top 0.203: ATMEL32U4.26 88.71,55.76 88.34,56.13 v87.83,56.13 | v79.07,46.73 75.77,46.73 75.51,46.48 v75.51,43.55
  Bottom 0.203: J4.2 75.47,43.51 v75.51,43.55 | v79.07,46.73 79.07,47.24 79.45,47.62 79.45,51.17 84.79,56.51 87.45,56.51 v87.83,56.13
D13  (via drill 0.2)
  Top 0.203: ATMEL32U4.32 85.71,54.06 85.42,54.35 82.75,54.35 82.5,54.6 v82.5,55.62 | v78.05,46.22 76.28,46.22 76.15,46.09 76.15,43.17 75.26,42.28 v74.75,42.28
  Bottom 0.203: J4.3 73.97,41.51 v74.75,42.28 | v82.5,55.62 82.5,55.49 78.44,51.43 78.44,48.13 78.05,47.75 v78.05,46.22
D+  (via drill 0.2)
  Top 0.203: v87.07,28.31 R2.1 86.42,30.35 86.18,30.35 85.8,30.73 Z2.1
  Bottom 0.203: J1.P3 87.71,27.68 v87.07,28.31
D-  (via drill 0.2)
  Top 0.203: v87.96,28.31 87.96,28.68 R3.1 89.63,30.35 89.74,30.35 90.25,30.85 Z1.1
  Bottom 0.203: J1.P2 88.37,27.91 v87.96,28.31
GND  (via drill 0.2)
  Top 0.203: ATMEL32U4.15 92.52,49.03 92.79,48.76 92.79,48.51 93.8,47.49 95.58,47.49 95.96,47.87 95.96,48.13 | ATMEL32U4.43 83.8,48.03 83.52,47.75 83.52,47.11 | ATMEL32U4.5 87.21,45.45 87.58,45.08
  other vias: 96.47,30.85 97.74,30.85 92.15,37.2 92.91,37.2 98.5,45.08 102.95,45.46 96.22,50.67 76.91,51.68 77.67,52.57 78.69,28.31 79.83,27.17 99.9,35.55 80.72,36.19 82.37,36.19 75.77,33.52 76.66,35.55 82.25,44.32 89.99,55.75 91.77,56.89 78.18,55.37 92.91,31.87 85.93,36.82 89.23,37.08 85.04,44.44 82.63,52.83 76.66,49.52 83.39,47.24 88.85,34.03 85.93,34.03 83.77,40 83.64,43.81 80.47,51.05 82.5,50.67 76.78,42.16 71.83,48.25 69.04,33.01 91.9,53.59 93.17,53.21 95.33,57.78 76.66,37.71 77.93,36.19 90.5,53.59 80.34,44.82
  pour Top (isolate 0.127, no thermals): 106.76,30.35 106.76,50.67 97.87,59.56 77.55,59.56 68.66,50.67 68.66,29.08 76.28,21.46 97.87,21.46
  pour Bottom (isolate 0.127, no thermals): 106.76,30.35 106.76,50.67 97.87,59.56 77.55,59.56 68.66,50.67 68.66,29.08 76.28,21.46 97.87,21.46
MISO
  Top 0.203: J2.1 96.09,41.65 94.69,42.92 93.29,42.92 93.04,43.17 93.04,44.19 91.01,46.22 90.62,46.22 ATMEL32U4.11
MOSI
  Top 0.203: ATMEL32U4.10 89.71,46.13 89.99,45.84 90.75,45.84 92.53,44.06 92.53,43.05 93.04,42.54 94.56,42.54 95.07,42.03 95.07,41.01 94.06,40 J2.5
N$1
  Top 0.254: ATMEL32U4.17 93.29,50.03 93.86,50.6 16M.1
N$2
  Top 0.254: ATMEL32U4.16 93.03,49.53 93.42,49.14 93.42,48.63 93.86,48.2 16M.3
N$3
  Top 0.203: IC4.1 96.6,34.45 96.6,33.52 95.71,32.63 92.66,32.63 92.15,32.12 92.15,29.2 92.53,28.82 92.53,26.28 91.77,25.52 90.25,25.52 89.74,25.01 89.74,24.38 89.36,24 CHG.C
N$4
  Top 0.203: R20.1 83.26,26.28 84.02,25.52 85.42,25.52 85.8,25.14 85.8,24.38 86.18,24 CHG.A
N$5  (via drill 0.2)
  Top 0.203: ATMEL32U4.6 v87.71,45.71 | C1.2 83.53,44.57 v83.64,44.57
  Bottom 0.203: v87.71,45.71 85.42,45.71 84.28,44.57 v83.64,44.57
N$6
  Top 0.203: ATMEL32U4.42 83.79,48.53 82.37,47.11 82.37,46.48 82.75,46.09 83.64,46.09 83.64,45.46 83.13,44.95 C2.2
N$7
  Top 0.203: TXD.A 89.88,58.4 90.63,57.65 90.63,57.02 91.52,56.13 93.04,56.13 93.29,56.38 R8.1
N$8
  Top 0.203: MCU6050.10 87.98,37.1 87.07,36.19 C4.1
N$9  (via drill 0.2)
  Top 0.203: MCU6050.20 88.49,43.32 88.72,43.55 v90.63,43.55 | C3.1 93.91,45.08 v92.91,45.08
  Bottom 0.203: v90.63,43.55 92.15,45.08 v92.91,45.08
N$10
  Top 0.203: R7.1 80.07,58.67 83.63,58.67 D7.A
N$11
  Top 0.203: ATMEL32U4.33 84.8,53.84 82.5,53.84 82.12,54.22 82.12,54.86 81.86,55.11 R1.2 81.61,55.11
N$12
  Top 0.203: T5.3 77.93,31.26 77.93,30.09 78.32,29.7 R18.2
N$13
  Top 0.203: R21.1 103.44,46.22 PWR.A
N$14
  Top 0.203: R12.2 95.83,53.84 96.09,53.59 96.09,53.33 96.85,52.57 T2.3
N$15
  Top 0.203: T1.3 78.84,49.68 79.2,50.03 R10.2
N$16  (via drill 0.36)
  Top 0.813: T1.1 v75.01,49.78
  Bottom 0.813: v75.01,49.78 74.52,49.27 69.55,49.27 69.42,49.4 arc36 JP1.P$1
N$17  (via drill 0.36)
  Top 0.813: T2.1 v99.62,50.69
  Bottom 0.813: v99.62,50.69 101.17,49.14 105.74,49.14 105.87,49.27 arc-33 JP3.P$1
N$18
  Top 0.203: R14.2 81.71,29.7 T3.3
N$19  (via drill 0.36)
  Top 0.813: T3.1 v80.75,24.28
  Bottom 0.813: v80.75,24.28 78.94,22.47 arc33 JP5.P$1
N$20
  Top 0.203: R16.2 95.68,29.7 T4.3
N$21  (via drill 0.36)
  Top 0.813: T4.1 v94.72,24.1
  Bottom 0.813: v94.72,24.1 96.47,22.35 arc-34 JP7.P$1
N$22
  Top 0.305: R19.1 76.01,31 74.63,32.38 T5.1
N$23  (via drill 0.2)
  Top 0.203: C9.1 85.91,34.78 86.18,35.05 v86.18,36.06
  Bottom 0.203: HMC5883.8 89.1,39.73 89.36,39.73 89.36,38.09 89.61,37.84 89.61,37.59 89.99,37.2 89.99,36.82 88.98,35.81 86.44,35.81 v86.18,36.06
N$24  (via drill 0.2)
  Top 0.254: LED7.C 63.42,10.79 arc-30 78.94,22.47 | 78.94,22.47 78.94,26.79 76.91,28.82 R19.2 76.04,29.7 73.74,32 71.2,32 69.55,33.65 69.55,49.27 arc28 58.12,64.92 LED4.C | LED6.C 111.99,10.79 111.33,10.79 arc33 96.34,22.47 | 96.34,22.47 78.94,22.47 | LED5.C 117.3,64.92 117.3,64.26 arc32 105.87,49.27 v105.87,47.87 | v104.98,37.97 104.34,37.33 104.34,36.44 105.99,34.79 105.99,32.89 105.23,32.12 101.3,32.12 96.72,27.55 96.72,25.27 96.34,24.89 96.34,22.47
  Bottom 0.254: v105.87,47.87 105.49,47.49 105.49,38.47 v104.98,37.97
N$25
  Bottom 0.203: U3.6 97.13,33.21 C6.1
N$26
  Top 0.203: R22.2 92.15,34.48 IC4.5
N$27
  Bottom 0.203: U3.4 97.13,35.11 C6.2
N$28  (via drill 0.2)
  Top 0.203: C9.2 v85.17,37.2
  Bottom 0.203: HMC5883.12 86.96,38.11 86.44,37.59 85.55,37.59 v85.17,37.2
N$29  (via drill 0.2)
  Top 0.203: v88.47,36.82 88.98,36.32 C10.1
  Bottom 0.203: HMC5883.10 87.96,37.34 v88.47,36.82
N$30  (via drill 0.36)
  Top 0.813: SW2.COM 101.8,41.27 101.04,40.51 v101.04,38.47 v101.04,37.59
  Bottom 0.813: VCC.1 v101.04,38.47
N$31
  Bottom 0.203: C11.1 80.89,32.51 83.26,32.51 83.87,33.11 U4.4
N$32  (via drill 0.2)
  Top 0.203: R23.1 v79.2,56.38 | D8.A 85.79,58.41 85.17,58.41 84.4,57.65 v82.25,57.65
  Bottom 0.203: v79.2,56.38 79.2,57.14 79.71,57.65 v82.25,57.65
N$34  (via drill 0.2)
  Top 0.203: T7.3 99.05,48.14 98.12,48.14 | 98.12,48.14 R24.2 | 98.12,48.14 v98.12,47.62
  Bottom 0.203: 98.16,47.65 v98.12,47.62 98.12,47.21 U7.4
N$35  (via drill 0.2)
  Top 0.203: R26.2 95.47,52.44 v96.09,52.44
  Bottom 0.203: v96.09,52.44 95.94,52.3 BT4.0.4
RESET  (via drill 0.2)
  Top 0.203: ATMEL32U4.13 91.61,48.03 91.9,47.75 91.9,46.35 92.41,45.84 v92.91,45.84
  Top 0.305: R4.1 93.29,46.22 v92.91,45.84
  Bottom 0.203: J2.3 92.02,42.03 93.55,43.55 93.55,45.21 v92.91,45.84
RX  (via drill 0.2)
  Top 0.203: ATMEL32U4.20 91.87,51.53 v92.41,52.06
  Bottom 0.203: BT4.0.2 93.17,54.1 92.53,53.46 92.53,52.19 v92.41,52.06
RXLED  (via drill 0.2)
  Top 0.203: ATMEL32U4.8 88.71,45.98 89.61,45.08 90.25,45.08 91.14,44.19 v91.14,42.92
  Bottom 0.203: v91.14,42.92 91.52,42.92 RXD.1
SCK
  Top 0.203: ATMEL32U4.9 89.21,45.99 89.74,45.46 90.5,45.46 92.02,43.94 92.02,42.92 93.42,41.52 J2.2
SCL  (via drill 0.2)
  Top 0.203: 86.94,43.3 v87.07,43.43 | v90.12,44.06 88.6,44.06 87.96,43.43 v87.07,43.43 | MCU6050.23 86.94,43.3 | 86.94,43.3 arc-90 v87.07,43.43 | v83.52,42.54 82.12,41.14 R6.1 | ATMEL32U4.18 92.91,50.53 v93.29,50.92
  Bottom 0.203: HMC5883.1 86.96,43.31 v87.07,43.43 85.8,43.43 84.91,42.54 v83.52,42.54 81.86,42.54 | v90.12,44.06 90.25,44.06 92.79,46.6 92.79,46.86 93.93,48 93.93,50.16 93.29,50.79 v93.29,50.92 | 81.86,42.54 80.09,42.54 78.56,41.01 78.56,40 77.55,38.98 75.39,38.98 74.86,39.51 J4.4 | BMP180.5 81.81,42.48 81.86,42.54
SDA  (via drill 0.2)
  Top 0.203: v85.85,42.59 MCU6050.24 86.44,43.81 86.56,43.94 87.83,43.94 88.47,44.57 v89.61,44.57 | ATMEL32U4.19 92.39,51.03 v92.79,51.43 | v83.52,41.27 82.12,39.87 R5.1 81.37,39.63 80.72,38.98 79.83,38.98 v79.2,38.35
  Bottom 0.203: BMP180.6 83.21,41.96 83.52,41.65 v83.52,41.27 85.55,41.27 | 85.55,41.27 86.32,41.27 HMC5883.16 | 85.55,41.27 85.6,41.32 85.6,42.33 v85.85,42.59 | v89.61,44.57 89.99,44.57 92.28,46.86 92.28,46.98 93.29,48 93.29,49.9 92.66,50.54 92.66,51.3 v92.79,51.43 | v79.2,38.35 73.55,38.35 J4.5
TX
  Top 0.203: ATMEL32U4.21 91.74,52.03 91.9,52.19 91.9,52.44 92.15,52.7 92.79,52.7 92.91,52.57 R26.1
TXLED
  Top 0.203: ATMEL32U4.22 91.14,52.56 91.14,55.75 89.98,56.9 TXD.C
USBD+  (via drill 0.2)
  Top 0.305: ATMEL32U4.4 86.71,45.19 v86.82,45.08 | v91.01,37.97 90.63,37.59 90.63,37.2 90.75,37.08 90.75,33.9 89.74,32.89 88.34,32.89 87.07,31.62 R2.2
  Bottom 0.305: v86.82,45.08 88.09,45.08 90.75,42.41 90.75,38.22 v91.01,37.97
USBD-  (via drill 0.2)
  Top 0.305: ATMEL32U4.3 86.21,45.23 v86.06,45.08 | v91.26,37.33 91.26,33.14 90.5,32.38 89.48,32.38 88.98,31.87 R3.2
  Bottom 0.305: v91.26,37.33 90.75,37.33 90.12,37.97 90.12,42.16 87.83,44.44 86.06,44.44 v86.06,45.08
VCC
  Top 0.406: IC4.3 101.1,36.38 102.69,37.97 SW2.A
VUSB  (via drill 0.2, 0.36)
  Top 0.203: ATMEL32U4.7 88.21,45.98 88.34,45.84 88.34,45.59 v88.72,45.21
  Top 0.305: ATMEL32U4.2 85.71,45.87 85.04,45.21 v84.15,45.21 84.28,45.08 84.28,44.06 84.66,43.68 84.66,38.6 84.4,38.35
  Top 0.406: 84.4,38.35 83.39,37.33 | 83.39,37.33 C17.2 | 83.39,37.33 83.26,37.2 R20.2 84.01,31 84.66,30.35 v84.66,28.95 | v91.52,28.44 91.52,32.38 92.41,33.27 94.69,33.27 95.33,33.9 95.33,35.43 94.38,36.38 IC4.4 94.03,36.92 95.2,38.09 98.88,38.09 100.15,39.36 100.15,41.65 99.64,42.16 99.64,44.7 101.42,46.48 T7.1
  Bottom 0.203: J1.P1 89.03,27.35 | v88.72,45.21 88.72,45.97 88.47,46.22 85.17,46.22 v84.15,45.21
  Bottom 0.406: 89.03,27.35 89.03,28.44 | v91.52,28.44 89.03,28.44 | 89.03,28.44 88.39,29.08 84.79,29.08 v84.66,28.95

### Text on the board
tPlace: Crazebird | R | S | I | SCL | SDA | G | MO | V | CH/NO | 3.3V | GND
bPlace: + | + | A1/A5 | D11 | D12 | D13 | BMP180 | SCL | SDA | CH/NO | 3.3V | GND | 15.5.25v0.5 | VCC | GND | + | +
tNames: VCC | GND | 2015/3/9-v1.0
bNames: GND

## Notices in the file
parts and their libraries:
SparkFun-DigitalIC: Licensing: CC v3.0 Share-Alike You are welcome to use this library for commercial purposes.
